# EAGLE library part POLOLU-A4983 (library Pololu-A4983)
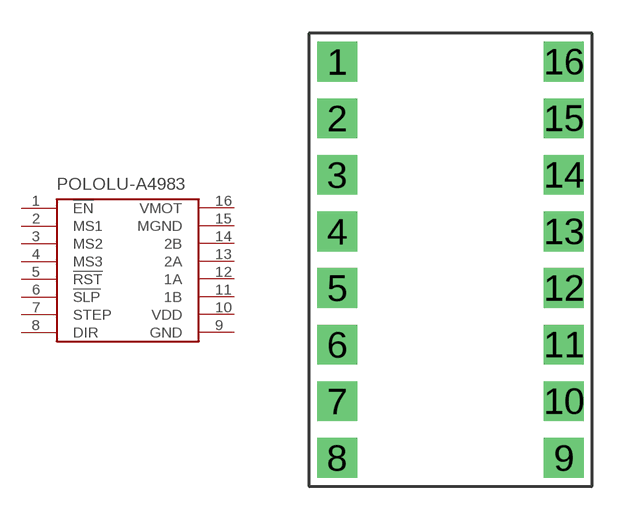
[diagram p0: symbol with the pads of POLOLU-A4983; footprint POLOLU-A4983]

Designator prefix -

## POLOLU-A4983POLOLU-A4983  [POLOLU-A4983]
1  !EN
2  MS1
3  MS2
4  MS3
5  !RST
6  !SLP
7  STEP
8  DIR
9  GND
10  VDD
11  1B
12  1A
13  2A
14  2B
15  MGND
16  VMOT

## Footprint POLOLU-A4983 (pad centres in mm)
drill 1 pad 1.778 square: 1 -5.08,8.89; 2 -5.08,6.35; 3 -5.08,3.81; 4 -5.08,1.27; 5 -5.08,-1.27; 6 -5.08,-3.81; 7 -5.08,-6.35; 8 -5.08,-8.89; 9 5.08,-8.89; 10 5.08,-6.35; 11 5.08,-3.81; 12 5.08,-1.27; 13 5.08,1.27; 14 5.08,3.81; 15 5.08,6.35; 16 5.08,8.89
